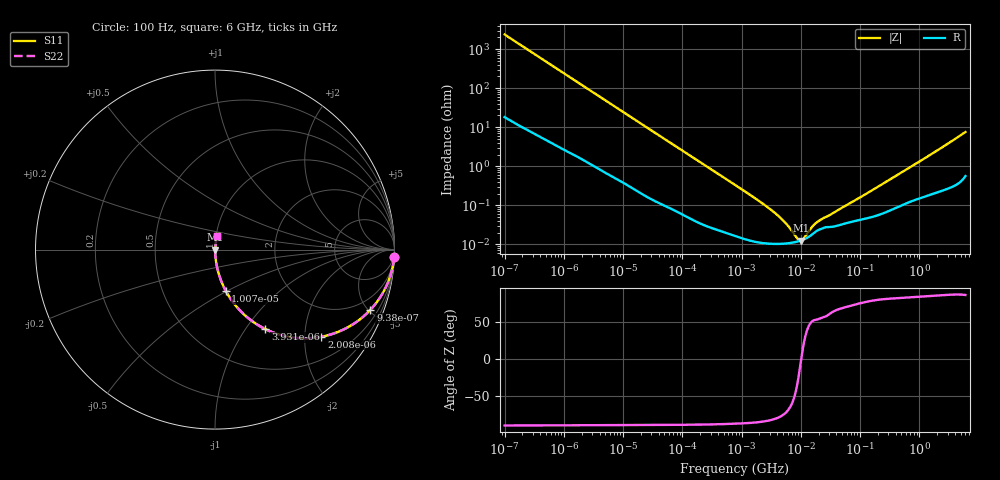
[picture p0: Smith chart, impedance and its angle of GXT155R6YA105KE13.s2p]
!Murata Part Number: GXT155R6YA105KE13
!These Parameters are Measured in Series Mode Connection
!Data Generated on Jan 08, 2026
!  o--ll--o
!Port1  Port2
!  o------o
!Operation Temp=25[degC], DC Bias Voltage=0[V]
!Freq. Start=100[Hz] Stop=6[GHz] 401[Steps]
# Hz S RI R 50
!Freq.(Hz) S11(Real) S11(Imag) S21(Real) S21(Imag) S12(Real) S12(Imag) S22(Real) S22(Imag)
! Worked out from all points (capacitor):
!   401 points, 100 Hz to 6 GHz, reference 50 ohm
!   read as one part in series: C = 666 nF near 109 Hz
!   lowest |Z| = 12.5 mohm at 9.942 MHz (marker M1)
!   series resonance near 10.18 MHz, so ESL is about 370 pH
!   S11 on the Smith chart (normalised r, x): 100 Hz: 1, -48; 938 Hz: 1.06, -5.14; 2.008 kHz: 1.03, -2.42; 3.931 kHz: 1.02, -1.24; 10.07 kHz: 1.01, -0.49; 6 GHz: 1.01, +0.15
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100  0.9979 -0.0419  0.00208 0.0419  0.00208 0.0419  0.9979 -0.0419
335  0.9797 -0.1367  0.0203 0.1367  0.0203 0.1367  0.9797 -0.1367
600  0.9395 -0.2335  0.0605 0.2335  0.0605 0.2335  0.9395 -0.2335
938  0.866 -0.3352  0.134 0.3352  0.134 0.3352  0.866 -0.3352
1342  0.762 -0.42  0.238 0.42  0.238 0.42  0.762 -0.42
2008  0.5925 -0.4851  0.4075 0.4851  0.4075 0.4851  0.5925 -0.4851
2748  0.4404 -0.49  0.5596 0.49  0.5596 0.49  0.4404 -0.49
3931  0.2809 -0.4427  0.7191 0.4427  0.7191 0.4427  0.2809 -0.4427
6151  0.1405 -0.3404  0.8595 0.3404  0.8595 0.3404  0.1405 -0.3404
10066  0.0596 -0.2291  0.9404 0.2291  0.9404 0.2291  0.0596 -0.2291
18841  0.019 -0.1287  0.981 0.1287  0.981 0.1287  0.019 -0.1287
40335  0.00493 -0.0615  0.9951 0.0615  0.9951 0.0615  0.00493 -0.0615
774597  0.000175 -0.00333  0.9998 0.00333  0.9998 0.00333  0.000175 -0.00333
3712478  0.000103 -0.000615  0.9999 0.000615  0.9999 0.000615  0.000103 -0.000615
5554849  0.000105 -0.000332  0.9999 0.000332  0.9999 0.000332  0.000105 -0.000332
8692127  0.000117 -8.14e-05  0.9999 8.14e-05  0.9999 8.14e-05  0.000117 -8.14e-05
9941735  0.000124 -1.19e-05  0.9999 1.19e-05  0.9999 1.19e-05  0.000124 -1.19e-05
1.137099e7  0.000134 5.71e-05  0.9999 -5.71e-05  0.9999 -5.71e-05  0.000134 5.71e-05
1.555665e7  0.00018 0.000217  0.9998 -0.000217  0.9998 -0.000217  0.00018 0.000217
2.225763e7  0.00025 0.000358  0.9997 -0.000358  0.9997 -0.000358  0.00025 0.000358
3.124326e8  0.000744 0.00445  0.9993 -0.00445  0.9993 -0.00445  0.000744 0.00445
6e9  0.0111 0.0741  0.9889 -0.0741  0.9889 -0.0741  0.0111 0.0741
